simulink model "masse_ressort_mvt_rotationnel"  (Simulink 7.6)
settings: Solver=ode15s  StartTime=0.0  StopTime=1  RelTol=1e-3
InitFcn:
  | J=0.01;
  | B=0.1;
  | k=10;
StopFcn:
  | % lecture du fichier binaire
  | load masse_ressort2.mat
  | 
  | % trace de la tension et du courant d’induit
  | plotyy(x(1,:),x(2,:),x(1,:),x(3,:))
  | title('Position et vitesse angulaires')
  | grid
libraries: fl_lib x6, nesl_utility x3

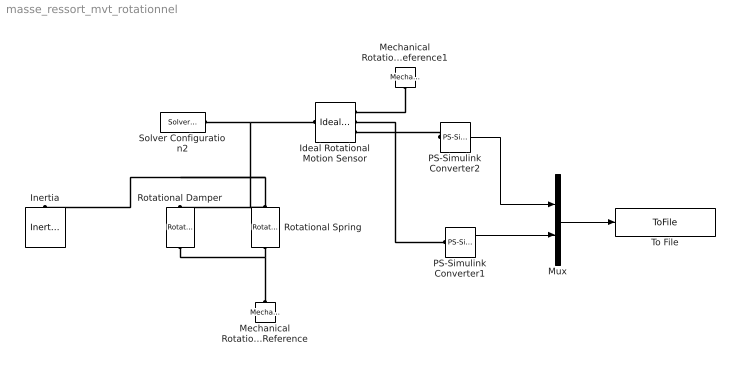
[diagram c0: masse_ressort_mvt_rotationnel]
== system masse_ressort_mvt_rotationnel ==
  Ideal Rotational Motion Sensor : fl_lib/Mechanical/Mechanical Sensors/Ideal Rotational Motion Sensor  DialogController=NetworkEngine.DynNeDlgSource  SystemSampleTime=-1  offset=0 rad  w_Log=off  t_Log=off  phi_Log=off  LocalVarNames=|w|t|phi  LocalVarDescs=|w|t|phi  LocalVarLogging=[0 0 0]
  Inertia : fl_lib/Mechanical/Rotational Elements/Inertia  DialogController=NetworkEngine.DynNeDlgSource  SystemSampleTime=-1  inertia=J kg*m^2  initial_velocity=10 rad/s  t_Log=off  LocalVarNames=|t  LocalVarDescs=|t  LocalVarLogging=0
  Mechanical Rotational Reference : fl_lib/Mechanical/Rotational Elements/Mechanical Rotational Reference  DialogController=NetworkEngine.DynNeDlgSource  SystemSampleTime=-1  t_Log=off  LocalVarNames=|t  LocalVarDescs=|t  LocalVarLogging=0
  Mechanical Rotational Reference1 : fl_lib/Mechanical/Rotational Elements/Mechanical Rotational Reference  DialogController=NetworkEngine.DynNeDlgSource  SystemSampleTime=-1  t_Log=off  LocalVarNames=|t  LocalVarDescs=|t  LocalVarLogging=0
  Mux : Mux  Inputs=2
  PS-Simulink Converter1 : nesl_utility/PS-Simulink Converter  DialogController=NetworkEngine.DynNeUtilDlgSource  SystemSampleTime=-1  PhysicalDomain=network_engine_domain  LeftPortType=input  RightPortType=output  SubClassName=ps_output  Unit=1  AffineConversion=off
  PS-Simulink Converter2 : nesl_utility/PS-Simulink Converter  DialogController=NetworkEngine.DynNeUtilDlgSource  SystemSampleTime=-1  PhysicalDomain=network_engine_domain  LeftPortType=input  RightPortType=output  SubClassName=ps_output  Unit=1  AffineConversion=off
  Rotational Damper : fl_lib/Mechanical/Rotational Elements/Rotational Damper  DialogController=NetworkEngine.DynNeDlgSource  SystemSampleTime=-1  D=B N*m/(rad/s)  t_Log=off  w_Log=off  LocalVarNames=|t|w  LocalVarDescs=|t|w  LocalVarLogging=[0 0]
  Rotational Spring : fl_lib/Mechanical/Rotational Elements/Rotational Spring  DialogController=NetworkEngine.DynNeDlgSource  SystemSampleTime=-1  spr_rate=k N*m/rad  init_def=0 rad  t_Log=off  w_Log=off  phi_Log=off  LocalVarNames=|t|w|phi  LocalVarDescs=|t|w|phi  LocalVarLogging=[0 0 0]
  Solver Configuration2 : nesl_utility/Solver Configuration  DialogController=NetworkEngine.DynNeUtilDlgSource  SystemSampleTime=-1  PhysicalDomain=network_engine_domain  LeftPortType=input  RightPortType=generic  SubClassName=solver  Accelerate=off  Profile=off  ResidualTolerance=1e-9  MaxNonlinIter=12  MaxModeIter=2  DoFixedCost=off  UseLocalSampling=off  DoDC=off  LinearAlgebra=Sparse  LocalSolverSampleTime=.001  LocalSolverChoice=NE_BACKWARD_EULER_ADVANCER  UseLocalSolver=off
  To File : ToFile  Filename=masse_ressort2.mat  MatrixName=x
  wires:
  PS-Simulink Converter2/1 -> Mux/1
  Mux/1 -> To File/1
  PS-Simulink Converter1/1 -> Mux/2
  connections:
  PS-Simulink Converter2/LConn1 -- Ideal Rotational Motion Sensor/RConn3
  Rotational Damper/RConn1 -- Mechanical Rotational Reference/LConn1 -- Rotational Spring/RConn1
  Ideal Rotational Motion Sensor/RConn2 -- PS-Simulink Converter1/LConn1
  Solver Configuration2/RConn1 -- Rotational Damper/LConn1 -- Inertia/LConn1 -- Rotational Spring/LConn1 -- Ideal Rotational Motion Sensor/LConn1
  Mechanical Rotational Reference1/LConn1 -- Ideal Rotational Motion Sensor/RConn1
